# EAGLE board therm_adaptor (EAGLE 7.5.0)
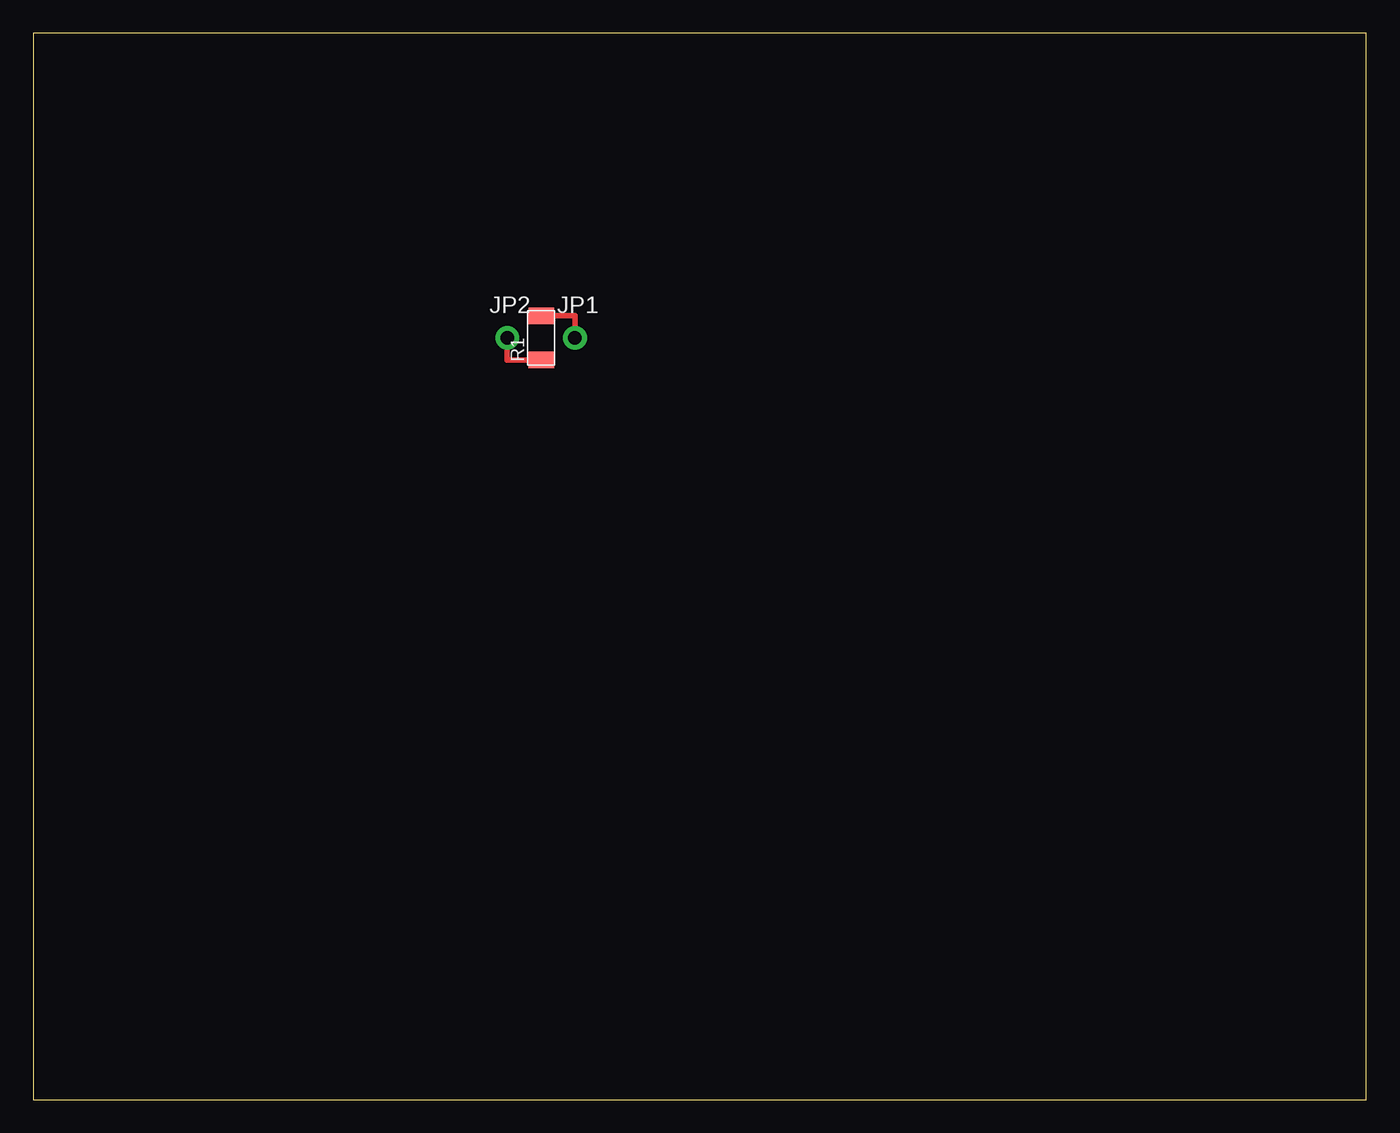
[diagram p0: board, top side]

Size 100 x 80 mm. Coordinates in mm from the lower left corner, seen from the top.
Outline: 0,0 100,0 100,80 0,80 0,0
Copper layers (1*16): Top 0.035mm / dielectric 1.5mm / Bottom 0.035mm
Design rules "default": minimum track width 10mil, minimum drill 24mil, track to track 8mil, track to pad 8mil, pad to pad 8mil, via to via 8mil, smd to smd 8mil, copper to edge 40mil, drill to drill 8mil, minimum pad ring 10mil, minimum via ring 8mil, stop-mask expansion 4mil, vias tented up to drill 0mil, thermal gap 10mil

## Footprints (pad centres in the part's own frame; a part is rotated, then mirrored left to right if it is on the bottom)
1X01-CLEANBIG = drill 1.016 pad 1.778: 1 0,0
R1206FAB = smd 1.27 x 1.905: 1 -1.651,0; 2 1.651,0

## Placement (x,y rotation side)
JP1  [1X01-CLEANBIG]  40.64,57.15 0 top
JP2  [1X01-CLEANBIG]  35.56,57.15 0 top
R1  [R1206FAB]  38.1,57.15 90 top

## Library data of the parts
JP1 JP2 = adafruit
R1 = 01fab

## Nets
N$1: JP2.1 R1.1
N$2: JP1.1 R1.2

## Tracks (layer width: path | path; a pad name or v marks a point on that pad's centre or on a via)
N$1
  Top 0.406: R1.1 35.56,55.5 JP2.1
N$2
  Top 0.406: R1.2 40.64,58.8 JP1.1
